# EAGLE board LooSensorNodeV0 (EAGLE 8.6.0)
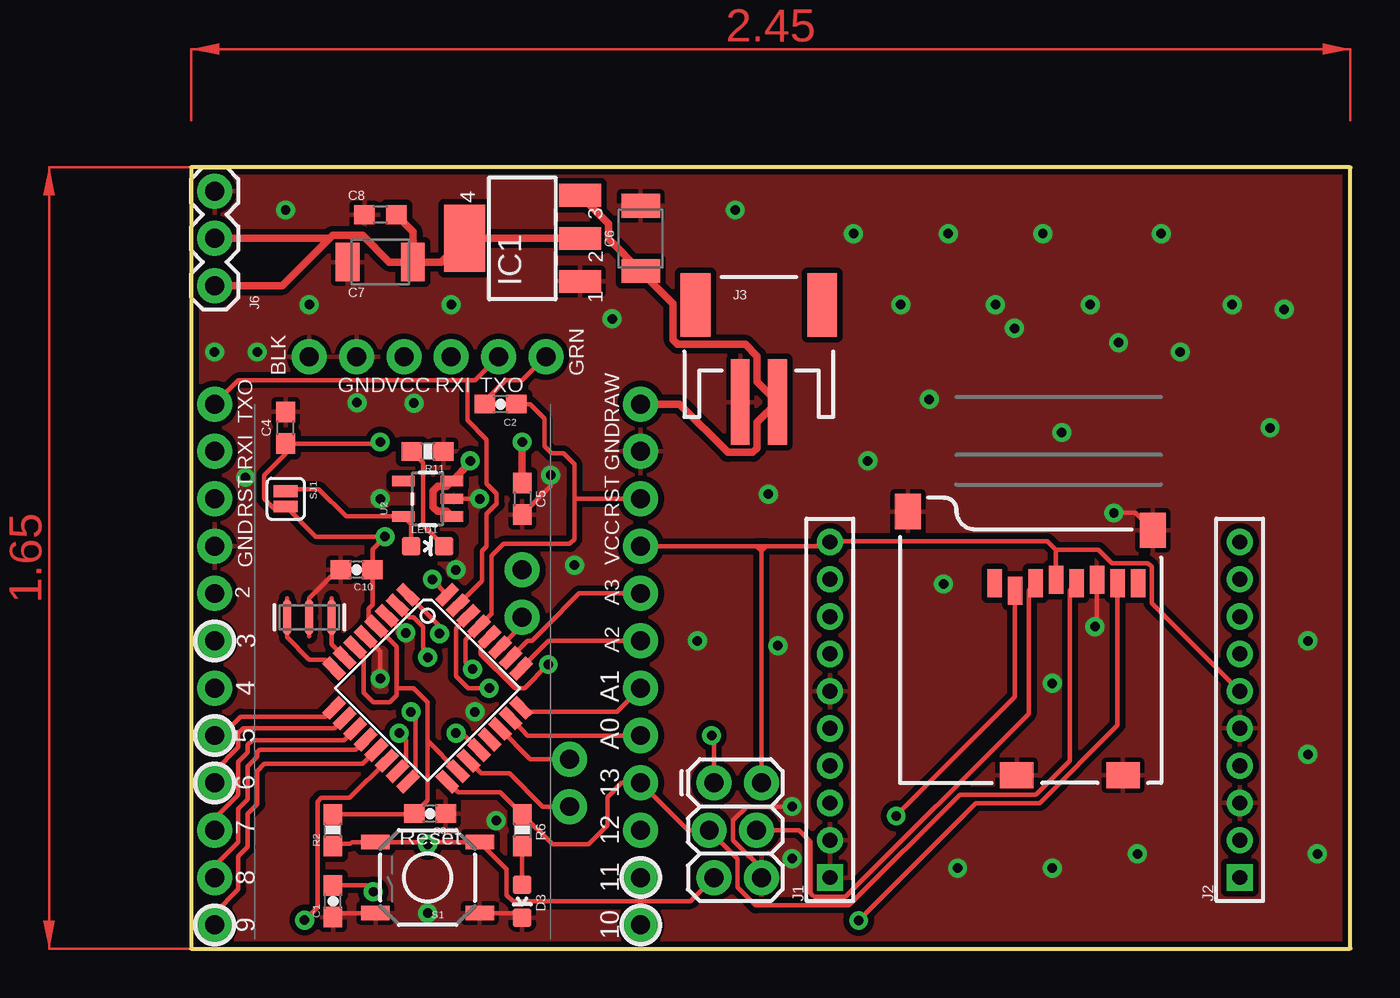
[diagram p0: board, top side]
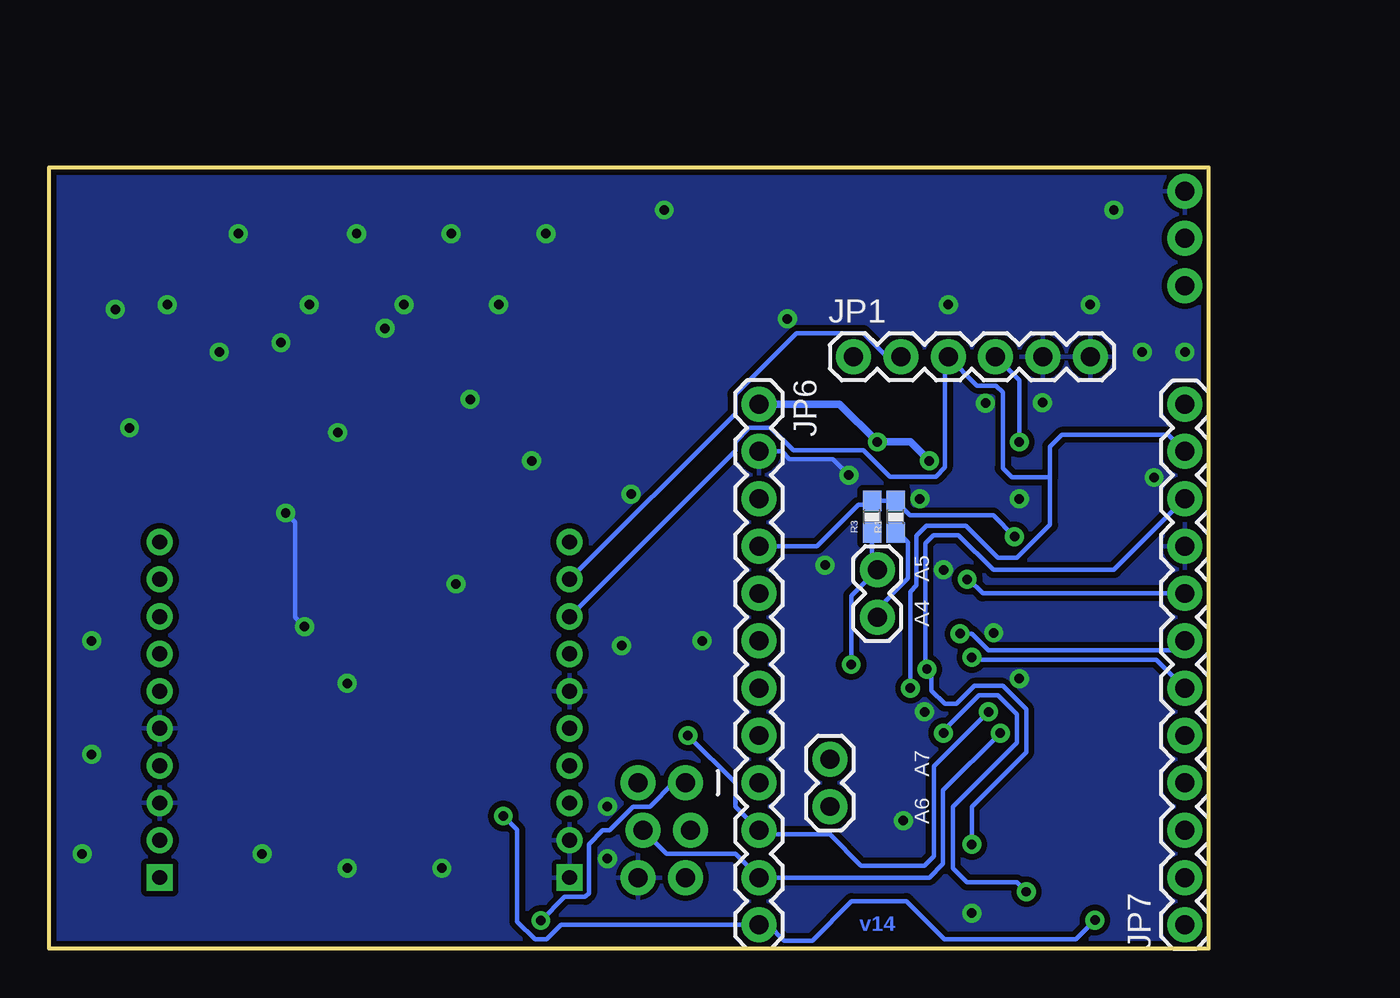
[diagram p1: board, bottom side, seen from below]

Size 62.23 x 41.91 mm. Coordinates in mm from the lower left corner, seen from the top.
Outline: 0,41.91 0,0 62.23,0 62.23,41.91 0,41.91
Copper layers (1*16): Top 0.035mm / dielectric 1.5mm / Bottom 0.035mm
Design rules "SparkFun-2-layer *": minimum track width 7mil, minimum drill 15mil, track to track 8mil, track to pad 8mil, pad to pad 8mil, via to via 8mil, smd to smd 8mil, copper to edge 8mil, drill to drill 8mil, minimum pad ring 12mil, minimum via ring 10mil, stop-mask expansion 4mil, vias tented up to drill 20mil, thermal gap 10mil
Net classes: 0 default: width 0.203 mm; 1 vcc: width 0.254 mm

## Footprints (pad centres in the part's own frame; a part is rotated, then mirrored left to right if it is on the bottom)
0603-CAP = smd 1.1 x 1: 1 -0.85,0; 2 0.85,0
0603 = smd 1.1 x 1: 1 -0.85,0; 2 0.85,0
1210 = smd 1.27 x 2.06: 1 -1.755,0; 2 1.755,0
0603-LED-ALT1 = smd 1 x 1: A 0,-0.877; C 0,0.877
SOT223 = smd 1.219 x 2.235: 1 -2.311,-3.099; 2 0,-3.099; 3 2.311,-3.099 | smd 3.6 x 2.2: 4 0,3.099
1X10-2MM = drill 0.8 square: 1 0,0 | drill 0.8: 2 2,0; 3 4,0; 4 6,0; 5 8,0; 6 10,0; 7 12,0; 8 14,0; 9 16,0; 10 18,0
JST-2-SMD = smd 1 x 4.6: 1 -1,-3.7; 2 1,-3.7 | smd 1.6 x 3.4: NC1 -3.4,1.5; NC2 3.4,1.5
2X3_LOCK = drill 1.016 pad 1.88: 1 0,0.127; 2 0,2.667; 3 2.54,-0.127; 4 2.54,2.413; 5 5.08,0.127; 6 5.08,2.667
MICRO-SD-SOCKET = smd 1.8 x 1.4: CD1 -2.05,0.4; CD2 -7.75,0.4 | smd 0.8 x 1.5: CS -7.84,10.3; DI -6.74,10.7; DO -2.34,10.7; GND -3.44,10.9; RSV1 -8.94,10.7; RSV2 -1.24,10.7; SCLK -4.54,10.7; VCC -5.64,10.9 | smd 1.4 x 1.9: GND1 -13.6,14.55; GND3 -0.45,13.55
1X03 = drill 1.016 pad 1.88: 1 0,0; 2 2.54,0; 3 5.08,0
1X06 = drill 1.016 pad 1.88: 1 0,0; 2 2.54,0; 3 5.08,0; 4 7.62,0; 5 10.16,0; 6 12.7,0
1X02 = drill 1.016 pad 1.88: 1 0,0; 2 2.54,0
1X12 = drill 1.016 pad 1.88: 1 0,0; 2 2.54,0; 3 5.08,0; 4 7.62,0; 5 10.16,0; 6 12.7,0; 7 15.24,0; 8 17.78,0; 9 20.32,0; 10 22.86,0; 11 25.4,0; 12 27.94,0
RESONATOR-SMD-1:1 = smd 0.45 x 1.905: 1 -1.2,0; 2 0,0; 3 1.2,0
0603-RES = smd 1.1 x 1: 1 -0.85,0; 2 0.85,0
TACTILE-SWITCH-SMD-ALT01 = smd 1.524 x 0.762: 1 -2.794,1.905; 2 2.794,1.905; 3 -2.794,-1.905; 4 2.794,-1.905
SJ_2S = smd 0.635 x 1.27: 1 -0.412,0; 2 0.412,0
TQFP32-08 = smd 1.27 x 0.559: 1 -4.293,2.8; 2 -4.293,2; 3 -4.293,1.2; 4 -4.293,0.4; 5 -4.293,-0.4; 6 -4.293,-1.2; 7 -4.293,-2; 8 -4.293,-2.8; 17 4.293,-2.8; 18 4.293,-2; 19 4.293,-1.2; 20 4.293,-0.4; 21 4.293,0.4; 22 4.293,1.2; 23 4.293,2; 24 4.293,2.8 | smd 0.559 x 1.27: 9 -2.8,-4.293; 10 -2,-4.293; 11 -1.2,-4.293; 12 -0.4,-4.293; 13 0.4,-4.293; 14 1.2,-4.293; 15 2,-4.293; 16 2.8,-4.293; 25 2.8,4.293; 26 2,4.293; 27 1.2,4.293; 28 0.4,4.293; 29 -0.4,4.293; 30 -1.2,4.293; 31 -2,4.293; 32 -2.8,4.293
SOT23-5 = smd 0.55 x 1.2: 1 -0.95,-1.3; 2 0,-1.3; 3 0.95,-1.3; 4 0.95,1.3; 5 -0.95,1.3

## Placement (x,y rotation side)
C1  0.1uF  [0603-CAP]  7.62,2.54 90 top
C2  0.1uF  [0603-CAP]  16.61,29.21 180 top
C3  0.1uF  [0603-CAP]  12.83,7.24 180 top
C4  10uF  [0603]  5.08,27.94 90 top
C5  10uF  [0603]  17.78,24.13 270 top
C6  47uF  [1210]  24.13,38.1 90 top
C7  47uF  [1210]  10.16,36.83 180 top
C8  0.1uF  [0603]  10.16,39.37 180 top
C10  0.1uF  [0603-CAP]  8.89,20.32 180 top
D3  Green  [0603-LED-ALT1]  17.78,2.54 180 top
FRAME1  FRAME-LETTER  [CREATIVE_COMMONS]  not placed on the board
IC1  MC33269ST-3.3T3  [SOT223]  17.78,38.1 90 top
J1  [1X10-2MM]  34.29,3.81 90 top
J2  [1X10-2MM]  56.29,3.81 90 top
J3  [JST-2-SMD]  30.48,33.02 0 top
J4  AVR_SPI_PROG_3X22X3_LOCK  [2X3_LOCK]  27.94,8.89 270 top
J5  MICRO-SD_CARD_SOCKET  [MICRO-SD-SOCKET]  52.07,8.89 0 top
J6  455-1750-1-ND  [1X03]  1.27,35.56 90 top
JP1  FTDI Basic  [1X06]  19.05,31.75 0 bottom
JP2  [1X02]  17.78,17.78 90 bottom
JP3  [1X02]  20.32,7.62 90 bottom
JP6  [1X12]  24.13,29.21 270 bottom
JP7  [1X12]  1.27,1.27 90 bottom
LED1  Red  [0603-LED-ALT1]  12.7,21.59 270 top
Q1  8/16/20MHz  [RESONATOR-SMD-1:1]  6.35,17.78 180 top
R1  [0603-RES]  16.79,23.16 90 bottom
R2  10K  [0603-RES]  7.62,6.35 90 top
R3  [0603-RES]  18.06,23.16 90 bottom
R6  330  [0603-RES]  17.78,6.35 270 top
R11  10K  [0603-RES]  12.7,26.67 180 top
S1  Reset  [TACTILE-SWITCH-SMD-ALT01]  12.7,3.81 180 top
SJ1  [SJ_2S]  5.08,24.13 270 top
U1  ATMEGA328  [TQFP32-08]  12.7,13.97 315 top
U2  MIC5205  [SOT23-5]  12.7,24.13 90 top

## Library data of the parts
C1-C3 C10 JP1-JP3 JP6 JP7 R1-R3 R6 R11 U1 U2 = SparkFun
C4 C5 = SparkFun-Capacitors; PROD_ID: CAP-11015
C6 C7 = SparkFun-Capacitors; PROD_ID: CAP-09824
C8 = SparkFun-Capacitors; PROD_ID: CAP-08604
D3 LED1 Q1 S1 = Testing
FRAME1 = SparkFun-Aesthetics
IC1 = linear
J1 J2 = SparkFun-Connectors; PROD_ID: CONN-08875; SF_ID: PRT-08272
J3 = SparkFun-Connectors; PROD_ID: CONN-11443; SF_ID: PRT-08612
J4 = SparkFun-Connectors
J5 = SparkFun-Connectors; PROD_ID: CONN-07820; SF_ID: PRT-00127
J6 = SparkFun-Connectors; PROD_ID: XXX-00000
SJ1 = SparkFun-Passives

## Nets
5V: C7.1 C8.1 IC1.2 IC1.4 J6.1 J6.2
A0: JP6.8 U1.23
A1: JP6.7 U1.24
A2: JP6.6 U1.25
A3: JP6.5 U1.26
A4: JP2.1 R1.1 U1.27
A5: JP2.2 R3.1 U1.28
A6: JP3.1 U1.19
A7: JP3.2 U1.22
AREF: C1.2 U1.20
D2: JP7.8 U1.32
D3: JP7.7 U1.1
D4: JP7.6 U1.2
D5: JP7.5 U1.9
D6: JP7.4 U1.10
D7: JP7.3 U1.11
D8: JP7.2 U1.12
D9: JP7.1 U1.13
D10: J5.CS JP6.12 U1.14
DTR: C2.2 JP1.1
GND [vcc]: C1.1 C3.1 C4.2 C5.2 C6.2 C7.2 C8.2 C10.2 D3.C IC1.1 J1.1 J1.2 J1.6 J2.3 J2.5 J3.1 J4.6 J5.CD1 J5.CD2 J5.GND J5.GND1 J5.GND3 J6.3 JP1.5 JP1.6 JP6.2 JP7.9 Q1.2 R11.1 S1.1 S1.2 U1.3 U1.5 U1.21 U2.2
MISO: J4.1 J5.DO JP6.10 U1.16
MOSI: J4.4 J5.DI JP6.11 U1.15
N$1: Q1.3 U1.8
N$2: Q1.1 U1.7
N$3: LED1.A SJ1.1 U2.5
N$4: LED1.C R11.2
N$7: D3.A R6.2
RAW [vcc]: C5.1 C6.1 IC1.3 J3.2 JP6.1 U2.1 U2.3
RESET: C2.1 J4.5 JP6.3 JP7.10 R2.1 S1.3 S1.4 U1.29
RXI: J1.8 JP1.3 JP7.11 U1.30
SCK: J4.3 J5.SCLK JP6.9 R6.1 U1.17
TXO: J1.9 JP1.2 JP7.12 U1.31
VCC: C3.2 C4.1 C10.1 J1.10 J2.6 J4.2 J5.VCC JP1.4 JP6.4 R1.2 R2.2 R3.2 SJ1.2 U1.4 U1.6 U1.18

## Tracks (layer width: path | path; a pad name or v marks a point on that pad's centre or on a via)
5V
  Top 0.406: IC1.2 IC1.4 13.41,36.83 C7.1 | C8.1 11.91,38.47 C7.1 | C7.1 10.64,36.83 9.21,38.27 7.6,38.27 7.43,38.1 | J6.2 7.43,38.1 | J6.1 4.89,35.56 7.43,38.1
A0
  Top 0.254: 18.07,11.43 JP6.8 | U1.23 17.8,11.7 18.07,11.43 | 18.07,11.43
A1
  Top 0.254: U1.24 17.71,12.77 17.78,12.7 22.86,12.7 JP6.7
A2
  Top 0.254: U1.25 19.2,16.51 JP6.6
A3
  Top 0.254: U1.26 18.07,16.51 18.31,16.51 19.05,17.25 19.05,17.27 20.83,19.05 JP6.5
A4
  Top 0.254: U1.27 17.4,16.97 | 17.4,16.97 | JP2.1 17.78,17.35 17.4,16.97
  Bottom 0.254: 16.79,22.46 16.13,21.8 16.13,21.08 16.13,19.86 17.78,18.21 JP2.1 | R1.1 16.79,22.46 | 16.79,22.46 16.84,22.52
A5  (via drill 0.51)
  Top 0.254: v19.18,15.24 17.91,13.97 17.4,13.97 17.27,14.1 17.25,14.1 15.54,15.8 15.54,16.25 U1.28 | U1.28
  Bottom 0.254: R3.1 18.06,20.6 JP2.2 19.18,18.92 v19.18,15.24
A6
  Top 0.254: JP3.1 18.88,7.62 17.1,9.4 15.57,9.4 U1.19
A7
  Top 0.254: JP3.2 18.21,10.16 | 18.21,10.16 | 18.21,10.16 U1.22
AREF  (via drill 0.51)
  Top 0.254: 14.55,11.56 v14.22,11.56 14.55,11.56 | U1.20 14.55,11.56 | v9.78,3.05 9.44,3.39 C1.2
  Bottom 0.254: v14.22,11.56 14.22,11.68 12.32,13.59 11.3,13.59 10.29,12.57 10.29,11.05 13.72,7.62 13.72,4.32 12.95,3.56 10.29,3.56 v9.78,3.05
D2  (via drill 0.51)
  Top 0.254: U1.32 12.95,19.79 v12.95,19.81
  Bottom 0.254: JP7.8 12.12,19.05 12.88,19.81 v12.95,19.81
D3  (via drill 0.51)
  Top 0.254: 13.34,17.3 v13.34,16.89 13.34,17.3 | U1.1 13.34,17.3
  Bottom 0.254: JP7.7 1.78,16 11.81,16 12.7,16.89 v13.34,16.89
D4  (via drill 0.51)
  Top 0.254: v12.7,15.62 12.95,15.62 12.45,16.13 12.45,17.27 11.94,17.78 11.72,17.78 | U1.2 11.72,17.78 | 11.72,17.78
  Bottom 0.254: JP7.6 2.79,15.49 12.57,15.49 v12.7,15.62
D5
  Top 0.254: JP7.5 1.65,11.43 2.67,12.45 7.22,12.45 U1.9
D6
  Top 0.254: 1.27,9.18 JP7.4 1.27,9.53 2.54,10.79 2.54,11.56 2.79,11.81 7.71,11.81 | U1.10 7.71,11.81 | 7.71,11.81
D7
  Top 0.254: JP7.3 1.27,6.99 2.54,8.26 2.54,10.03 3.05,10.54 3.05,10.92 3.3,11.18 8.21,11.18 U1.11
D8
  Top 0.254: JP7.2 1.27,4.45 2.54,5.71 2.54,7.49 3.05,8 3.05,9.78 3.56,10.29 3.56,10.54 3.68,10.67 8.83,10.67 U1.12
D9
  Top 0.254: JP7.1 1.27,1.91 2.54,3.17 2.54,4.95 3.05,5.46 3.05,7.24 3.56,7.75 3.56,9.53 3.94,9.91 9.2,9.91 U1.13
D10  (via drill 0.51)
  Top 0.254: v6.1,1.52 6.79,2.22 6.79,7.89 6.98,8.08 8.51,8.08 U1.14 | J5.CS 44.23,13.5 v37.85,7.11
  Bottom 0.254: v6.1,1.52 7.11,0.51 14.19,0.51 16.22,2.54 19.15,2.54 21.26,0.43 22.78,0.43 23.62,1.27 JP6.12 34.74,1.27 35.52,0.49 36.15,0.49 37.1,1.44 37.1,6.37 v37.85,7.11
DTR
  Top 0.254: JP1.1 17.78,30.48 16.89,30.48 15.76,29.35 C2.2
GND  (via drill 0.51)
  Top 0.254: v15.49,24.13 13.97,24.13 | U1.3 11.48,16.89 11.56,16.89 | C1.1 7.83,1.91 S1.2 | U1.5 10.16,15.94 v10.16,14.48 | D3.C 17.54,1.91 S1.1 | Q1.2 6.35,18.8 7.87,20.32 C10.2 | J4.6 30.61,4.3 29.08,5.82 29.08,6.88 29.83,7.62 v32.26,7.62 | J5.GND 48.63,17.39 v48.51,17.27 | v49.53,23.37 50.69,23.37 J5.GND3 | C5.2 19.3,24.8 v19.3,25.4
  Bottom 0.254: v48.51,17.27 49.02,17.78 49.02,22.86 v49.53,23.37 | v19.3,25.4 20.17,26.26 22.48,26.26 22.88,26.67 JP6.2
  other vias: 15.24,12.7 12.7,1.91 8.92,29.29 14.22,20.32 11.53,16.94 2.92,25.27 10.16,24.13 11.96,29.26 16.38,6.86 20.57,20.57 41.15,4.32 50.8,5.08 30.99,24.38 31.5,16.26 27.18,16.51 46.23,14.22 40.39,19.56 36.32,26.16 46.23,4.32 60.45,5.08 59.94,10.41 59.94,16.51 39.62,29.46 44.2,33.27 53.09,32 46.74,27.69 57.91,27.94 58.67,34.29 49.78,32.51 38.1,34.54 22.61,33.78 3.56,32 32.26,4.83 35.56,38.35 40.64,38.35 43.18,34.54 45.72,38.35 48.26,34.54 52.07,38.35 55.88,34.54 29.21,39.62 13.97,34.54 5.08,39.62 1.27,32 6.35,34.54
  pour Top (isolate 0.305): -3.81,45.72 64.77,45.72 64.77,0 -3.81,0
  pour Bottom (isolate 0.305): 0,44.45 63.5,44.45 63.5,0 0,0
MISO  (via drill 0.51)
  Top 0.254: U1.16 12.06,9.38 12.06,12.45 v11.81,12.7 | J4.1 28.07,11.3 v27.94,11.43 | v35.83,1.5 42.13,7.8 45.55,7.8 49.73,11.99 J5.DO
  Bottom 0.254: v11.81,12.7 14.73,9.78 14.73,4.95 15.24,4.45 18.64,4.45 20.32,6.12 23.9,6.12 JP6.10 25.4,7.62 25.4,8.89 v27.94,11.43 | v35.83,1.5 34.56,2.77 33.45,2.77 33.26,2.97 33.26,5.61 32.51,6.35 32.15,6.35 30.88,7.62 29.97,7.62 28.7,8.89 J4.1
MOSI  (via drill 0.51)
  Top 0.254: v11.18,11.56 11.56,11.18 11.56,10 U1.15 | J5.DI 44.96,19.22 44.96,12.6 35.13,2.77 33.45,2.77 33.35,2.87 33.26,2.97 33.26,5.73 32.64,6.35 J4.4
  Bottom 0.254: v11.18,11.56 14.25,8.48 14.25,4.55 14.99,3.81 JP6.11 25.4,5.08 29.08,5.08 J4.4
N$1
  Top 0.254: Q1.3 5.15,16.69 6.35,15.49 7.22,15.49 U1.8
N$2
  Top 0.254: 7.97,15.87 U1.7 8.25,15.63 7.55,16.33 Q1.1
N$3
  Top 0.254: SJ1.1 5.18,24.64 6.86,24.64 8.32,23.18 U2.5 11.82,22.76 LED1.A
N$4
  Top 0.254: R11.2 12.45,26.07 12.45,22.72 LED1.C
N$7
  Top 0.254: D3.A R6.2
RAW  (via drill 0.51)
  Top 0.254: U2.3 14,25.13 14.02,25.15
  Top 0.406: IC1.3 22.4,38.88 22.4,38.07 C6.1 25.87,34.6 25.87,32.65 26.11,32.41 29.76,32.41 30.39,31.79 30.39,30.41 J3.2 30.39,28.23 30.39,26.85 30.15,26.61 28.81,26.61 26.21,29.21 JP6.1 | U2.1 13.73,23.45 13.23,23.45 12.99,23.69 12.99,24.57 13.23,24.81 13.73,24.81 U2.3 14.99,26.07 v14.99,26.16 | C5.1 v17.78,27.18
  Bottom 0.406: v14.99,26.16 16,27.18 v17.78,27.18 19.81,29.21 JP6.1
RESET  (via drill 0.51)
  Top 0.254: 20.57,24.13 JP6.3 | 20.57,24.13 20.57,21.97 20.32,21.72 16.76,21.72 16.13,21.08 16.13,17.96 U1.29 | v15.11,14.99 14.73,15.37 14.73,16.57 U1.29 | C2.1 18.19,29.21 18.97,28.42 18.97,26.95 19.36,26.56 19.99,26.56 20.57,25.97 20.57,24.13 | R2.1 7.74,5.62 8.54,5.62 8.64,5.71 S1.4 12.57,5.71 v12.7,5.59 12.83,5.71 S1.3 16.95,4.26 16.95,2.87 17.28,2.54 26.8,2.54 J4.5 | U1.29
  Bottom 0.254: v12.7,5.59 12.7,7.62 9.78,10.54 9.78,12.83 11.05,14.1 12.57,14.1 13.53,13.14 14.16,13.14 14.86,13.84 14.86,14.73 v15.11,14.99 15.19,15.06 15.19,21.74 14.76,22.17 13.41,22.17 11.56,20.32 5.08,20.32 JP7.10
RXI  (via drill 0.51)
  Top 0.254: v16,13.97 14.86,13.97 14.22,14.61 14.22,17.19 U1.30 | U1.30
  Bottom 0.254: v16,13.97 16,19.15 15.67,19.48 15.67,22.15 15.14,22.68 13.03,22.68 11.3,20.95 10.29,20.95 8.51,22.73 8.51,25.27 | JP7.11 2.16,27.56 7.87,27.56 8.51,26.92 8.51,25.27 | 8.51,25.27 10.54,25.27 11.05,25.78 11.05,29.84 11.4,30.2 12.42,30.2 JP1.3 14.15,31.57 14.15,25.82 14.64,25.32 17.11,25.32 18.51,26.72 22.29,26.72 23.51,27.94 24.66,27.94 25.4,27.2 25.4,26.7 J1.8
SCK
  Top 0.254: U1.17 14.33,8.38 16.6,8.38 R6.1 19.39,5.59 21.34,5.59 22.35,6.6 22.35,8.13 23.11,8.89 JP6.9 26.67,6.35 J4.3 29.34,4.83 29.34,3.28 30.3,2.32 35.32,2.32 41.26,8.26 45.36,8.26 47.16,10.06 47.16,19.22 J5.SCLK
TXO
  Top 0.254: JP7.12 2.54,30.48 14.83,30.48 | 14.83,30.48 15.24,30.48 JP1.2 | 15.62,19.72 15.62,21.34 15.88,21.59 15.88,23.32 16.41,23.85 16.41,24.41 15.88,24.94 15.88,27.3 14.83,28.35 14.83,30.48 | U1.31 15.62,19.72 | 15.62,19.72
  Bottom 0.254: J1.9 25.4,28.7 25.4,29.74 22.12,33.02 18.52,33.02 17.25,31.75 JP1.2
VCC  (via drill 0.51)
  Top 0.254: 12.7,11.14 12.75,11.1 12.7,11.05 | 12.7,11.05 12.7,11.14 | 12.7,11.14 12.7,13.21 11.94,13.97 11.05,13.97 | 11.05,13.97 11.05,13.59 10.67,13.21 9.78,13.21 9.27,13.72 9.27,15.7 U1.6 | 11.05,13.97 11.05,16.19 U1.4 | 12.7,11.05 12.7,7.96 C3.2 11.94,7.2 R2.2 | U1.18 12.7,11.14 | 9.95,17.31 U1.4 | v10.16,27.18 10.07,27.09 C4.1 5.08,26.54 3.94,25.4 3.94,24.13 4.45,23.62 5.18,23.62 SJ1.2 6.7,22.1 v10.41,22.1 9.74,21.42 C10.1 9.74,18.45 9.54,18.24 9.54,17.7 U1.4 | JP6.4 30.35,21.59 | 30.35,21.59 30.48,21.59 | 30.48,21.59 30.73,21.59 | 30.73,21.59 30.86,21.59 | 30.86,21.59 34.07,21.59 J1.10 34.32,21.84 45.97,21.84 46.43,21.39 | J4.2 30.61,21.34 | 30.61,21.34 30.61,21.46 | 30.61,21.46 30.73,21.59 | 30.61,21.46 30.48,21.59 | 30.61,21.34 30.86,21.59 | 30.61,21.34 30.35,21.59 | J5.VCC 46.43,21.39 | 46.43,21.39 48.71,21.39 49.43,20.67 51.37,20.67 51.56,20.48 51.56,18.54 J2.6
  Bottom 0.254: v10.16,27.18 10.16,30.48 JP1.4 | JP6.4 21.01,21.59 18.8,23.8 18.27,23.8 R3.2 R1.2 16.02,23.24 11.56,23.24 v10.41,22.1
(copper drawn outside any net)
  shapes: Top area x2

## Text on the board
Bottom: v14
tPlace: BLK | GRN | GND | VCC | RXI | TXO | TXO | RAW | RXI | GND | RST | RST | VCC | GND | 2 | A3 | 3 | A2 | 4 | A1 | 5 | A0 | 6 | 13 | 7 | Reset | 12 | 8 | 11 | 9 | 10
bPlace: A5 | A4 | A7 | A6
tValues: Arduino Pro Mini
tDocu: Original Arduino Mini Design by Team Arduino / Arduino Pro Mini Design by SparkFun Electronics / Revised by Pete Lewis / Revised by Brandon Ng

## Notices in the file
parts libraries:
SparkFun-Aesthetics: Licensing: CC v3.0 Share-Alike You are welcome to use this library for commercial purposes.
SparkFun-Aesthetics: Released under the Creative Commons Attribution Share-Alike 3.0 License
SparkFun-Aesthetics: http://creativecommons.org/licenses/by-sa/3.0
